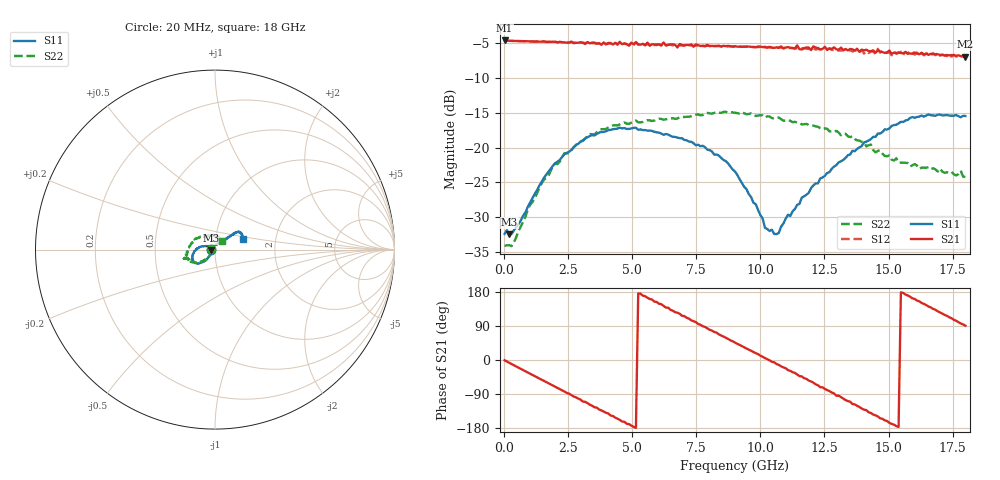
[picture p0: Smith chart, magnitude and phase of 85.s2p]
!Agilent Technologies,N5230A,US43500223,A.07.50.48
!Agilent N5230A: A.07.50.48
!Date: Monday, February 01, 2016 15:57:56
!Correction: S11(Full 2 Port(1,2))
!S21(Full 2 Port(1,2))
!S12(Full 2 Port(1,2))
!S22(Full 2 Port(1,2))
!S2P File: Measurements: S11, S21, S12, S22:
# Hz S  RI  R 50
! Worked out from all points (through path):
!   201 points, 20 MHz to 18 GHz, reference 50 ohm
!   highest |S21| = -4.61 dB at 20 MHz (marker M1); lowest = -6.9 dB at 18 GHz (marker M2)
!   group delay of S21, straight-line fit = 96.9 ps
!   lowest |S11| = -32.4 dB at 199.8 MHz (marker M3), VSWR 1.05, Z = 47.7 - j0.355 ohm
!   |S11| at or under -10 dB: start of sweep to end of sweep
!   |S22| runs from -34.1 to -14.8 dB; largest |S21 - S12| = 0.032
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2e7  -0.0241 0.000447  0.588 -0.00748  0.587 -0.00836  -0.0197 0.000939
1.998e8  -0.0236 -0.00372  0.5795 -0.0746  0.5797 -0.0754  -0.0197 -0.00343
9.19e8  -0.0258 -0.027  0.4877 -0.3146  0.4868 -0.3153  -0.0244 -0.026
1.818e9  -0.0448 -0.0545  0.2489 -0.5176  0.2441 -0.5209  -0.0472 -0.0491
3.0766e9  -0.0846 -0.075  -0.1903 -0.532  -0.1858 -0.5365  -0.088 -0.0691
4.515e9  -0.1218 -0.0674  -0.5287 -0.2136  -0.5341 -0.2153  -0.1309 -0.0664
5.1443e9  -0.1283 -0.0536  -0.5693 -0.00955  -0.5733 -0.00609  -0.1431 -0.0632
6.0433e9  -0.1248 -0.0296  -0.4711 0.2888  -0.4629 0.2978  -0.1524 -0.0522
7.4817e9  -0.104 0.000844  -0.0954 0.5417  -0.0764 0.5349  -0.1644 -0.052
8.2009e9  -0.0884 0.0115  0.148 0.5141  0.1537 0.5151  -0.1701 -0.0513
9.01e9  -0.0653 0.0172  0.3725 0.3845  0.3733 0.3778  -0.1707 -0.0513
1.01787e10  -0.0158 0.0214  0.5276 0.0478  0.5229 0.04  -0.1597 -0.0392
1.05383e10  -0.0049 0.0235  0.5176 -0.0546  0.5203 -0.0701  -0.158 -0.0331
1.20666e10  0.0333 0.0419  0.2684 -0.461  0.2436 -0.4552  -0.1425 0.0194
1.26959e10  0.0433 0.0507  0.0705 -0.509  0.046 -0.5158  -0.1253 0.0379
1.3505e10  0.066 0.0604  -0.1756 -0.4804  -0.1919 -0.464  -0.103 0.0597
1.45838e10  0.0962 0.0818  -0.4276 -0.2584  -0.4425 -0.2577  -0.056 0.0765
1.50333e10  0.1046 0.0892  -0.4826 -0.122  -0.4702 -0.1052  -0.0375 0.0794
1.58424e10  0.1288 0.1007  -0.4628 0.1067  -0.4822 0.1089  -0.00268 0.0732
1.64717e10  0.1414 0.0948  -0.3876 0.2719  -0.3919 0.2664  0.0168 0.0698
1.73707e10  0.1546 0.071  -0.1779 0.4239  -0.1654 0.4394  0.0335 0.0568
1.8e10  0.1588 0.057  -0.00404 0.4498  0.016 0.4517  0.0403 0.0469
